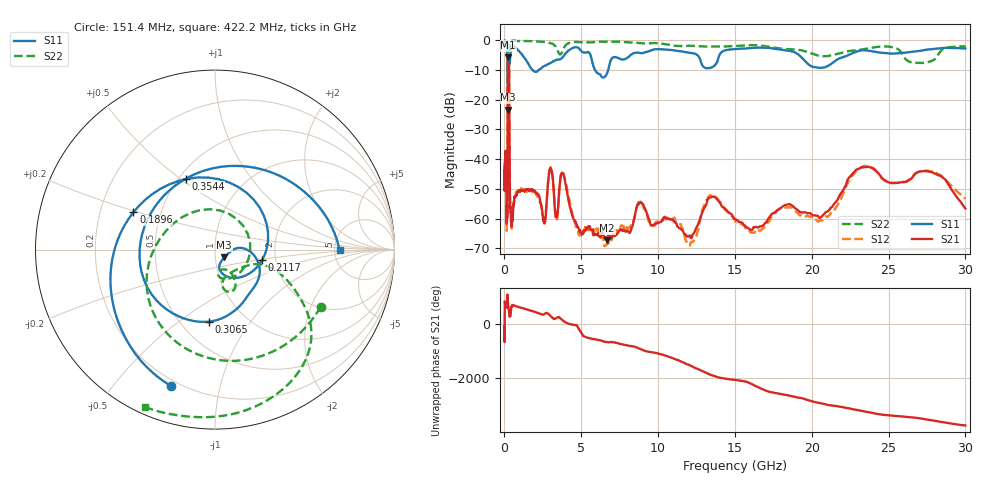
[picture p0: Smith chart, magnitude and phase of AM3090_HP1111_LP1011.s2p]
! Date/Time: Thu, Feb 28, 2019 2:10 PM
! Network Analyzer: Agilent Technologies E8364B Rev: A.07.50.67
! Sweep from 0.010 to 30.000 GHz, 1601 Points, Sweep Type: LOG
! Power Supply: 5.023 V, 0.002 A
# Hz S DB R 50
!freq MagS11 AngS11 MagS21 AngS21 MagS12 AngS12 MagS22 AngS22
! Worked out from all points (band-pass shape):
!   1601 points, 10 MHz to 30 GHz, reference 50 ohm
!   highest |S21| = -5.76 dB at 249.7 MHz (marker M1); lowest = -67.3 dB at 6.686 GHz (marker M2)
!   |S21| within 3 dB of the highest: 217.9 MHz to 293.4 MHz (75.47 MHz wide, 29.5 % of centre)
!   lowest |S11| = -23.4 dB at 239.9 MHz (marker M3), VSWR 1.15, Z = 55.2 - j4.83 ohm
!   |S11| at or under -10 dB: 206.9 MHz to 282.2 MHz (75.29 MHz wide, 30.8 % of centre); 1.813 GHz to 2.238 GHz (425.1 MHz wide, 21 % of centre); 5.885 GHz to 6.756 GHz (870.6 MHz wide, 13.8 % of centre)
!   |S22| runs from -18.6 to -0.2 dB; largest |S21 - S12| = 0.013
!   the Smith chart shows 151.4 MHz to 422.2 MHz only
!   S11 on the Smith chart (normalised r, x): 151.4 MHz: 0.17, -0.72; 189.6 MHz: 0.35, +0.19; 211.7 MHz: 1.70, -0.21; 306.5 MHz: 0.68, -0.65; 354.4 MHz: 0.54, +0.52; 422.2 MHz: 5.55, -0.09
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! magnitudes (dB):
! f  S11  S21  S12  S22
! 10 MHz  -0.3  -48.9  -41.6  -0.7
! 38.04 MHz  -0.3  -40.8  -41.2  -1.3
! 106.1 MHz  -1.0  -40.3  -39.9  -3.2
! 144.7 MHz  -1.7  -59.5  -59.5  -3.5
! 151.4 MHz  -2.0  -60.3  -64.1  -3.5
! 189.6 MHz  -6.0  -49.0  -48.1  -9.0
! 211.7 MHz  -11.4  -12.0  -11.9  -15.3
! 239.9 MHz  -23.4  -5.9  -5.9  -14.6
! 249.7 MHz  -19.5  -5.8  -5.7  -13.0
! 306.5 MHz  -7.9  -14.2  -14.1  -7.6
! 354.4 MHz  -7.4  -54.1  -51.5  -0.8
! 422.2 MHz  -3.2  -59.0  -58.5  -0.4
! 550.5 MHz  -2.0  -58.4  -56.5  -0.3
! 2.084 GHz  -10.7  -51.6  -51.8  -0.5
! 3.017 GHz  -7.6  -43.1  -42.8  -1.1
! 3.402 GHz  -6.6  -59.5  -60.6  -2.9
! 3.798 GHz  -5.8  -44.9  -44.3  -3.5
! 6.686 GHz  -11.1  -67.3  -68.3  -0.6
! 7.926 GHz  -6.2  -64.3  -63.8  -0.8
! 16.37 GHz  -2.6  -62.7  -63.6  -1.8
! 23.48 GHz  -3.5  -42.6  -42.3  -3.0
! 30 GHz  -2.9  -56.6  -53.3  -2.1
